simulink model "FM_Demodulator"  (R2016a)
settings: Solver=ode3  StartTime=0.0  StopTime=6  FixedStep=1/5000000  RelTol=1e-3
libraries: dsparch4 x4

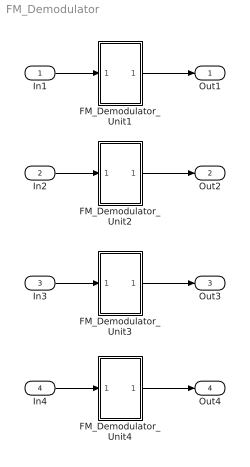
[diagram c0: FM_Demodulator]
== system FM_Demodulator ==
  In1 : Inport
  In2 : Inport  Port=2
  In3 : Inport  Port=3
  In4 : Inport  Port=4
  FM_Demodulator_Unit1 : Subsystem
  FM_Demodulator_Unit2 : Subsystem
  FM_Demodulator_Unit3 : Subsystem
  FM_Demodulator_Unit4 : Subsystem
  Out1 : Outport
  Out2 : Outport  Port=2
  Out3 : Outport  Port=3
  Out4 : Outport  Port=4
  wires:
  In1/1 -> FM_Demodulator_Unit1/1(In1)
  FM_Demodulator_Unit1/1(Out1) -> Out1/1
  In2/1 -> FM_Demodulator_Unit2/1(In1)
  FM_Demodulator_Unit2/1(Out1) -> Out2/1
  In3/1 -> FM_Demodulator_Unit3/1(In1)
  FM_Demodulator_Unit3/1(Out1) -> Out3/1
  In4/1 -> FM_Demodulator_Unit4/1(In1)
  FM_Demodulator_Unit4/1(Out1) -> Out4/1

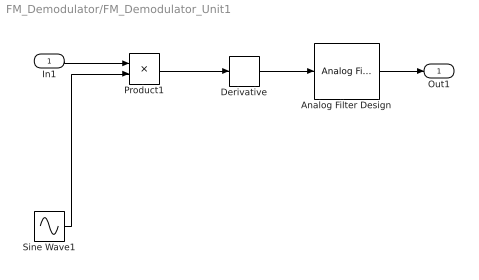
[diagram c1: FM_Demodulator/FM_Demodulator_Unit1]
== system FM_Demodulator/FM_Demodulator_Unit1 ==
  In1 : Inport
  Analog Filter Design : dsparch4/Analog Filter Design  method=Butterworth  filttype=Lowpass  N=10  Wlo=45000*2*pi  Whi=80  Rp=2  Rs=40
  Derivative : Derivative
  Product1 : Product
  Sine Wave1 : Sin  Frequency=500000*2*pi  Phase=-1.5*pi
  Out1 : Outport
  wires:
  Analog Filter Design/1 -> Out1/1
  Product1/1 -> Derivative/1
  Sine Wave1/1 -> Product1/2
  In1/1 -> Product1/1
  Derivative/1 -> Analog Filter Design/1

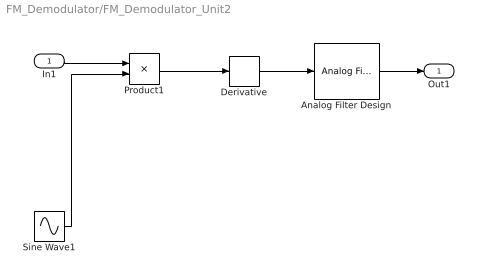
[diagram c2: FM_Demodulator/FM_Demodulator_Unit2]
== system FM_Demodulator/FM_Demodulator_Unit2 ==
  In1 : Inport
  Analog Filter Design : dsparch4/Analog Filter Design  method=Butterworth  filttype=Lowpass  N=10  Wlo=45000*2*pi  Whi=80  Rp=2  Rs=40
  Derivative : Derivative
  Product1 : Product
  Sine Wave1 : Sin  Frequency=500000*2*pi  Phase=-1.5*pi
  Out1 : Outport
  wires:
  Analog Filter Design/1 -> Out1/1
  Product1/1 -> Derivative/1
  Sine Wave1/1 -> Product1/2
  In1/1 -> Product1/1
  Derivative/1 -> Analog Filter Design/1

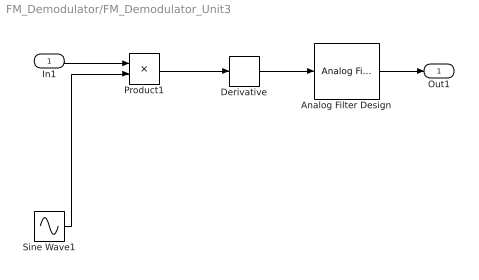
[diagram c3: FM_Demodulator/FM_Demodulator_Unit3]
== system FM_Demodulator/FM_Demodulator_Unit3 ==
  In1 : Inport
  Analog Filter Design : dsparch4/Analog Filter Design  method=Butterworth  filttype=Lowpass  N=10  Wlo=45000*2*pi  Whi=80  Rp=2  Rs=40
  Derivative : Derivative
  Product1 : Product
  Sine Wave1 : Sin  Frequency=500000*2*pi  Phase=-1.5*pi
  Out1 : Outport
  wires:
  Analog Filter Design/1 -> Out1/1
  Product1/1 -> Derivative/1
  Sine Wave1/1 -> Product1/2
  In1/1 -> Product1/1
  Derivative/1 -> Analog Filter Design/1

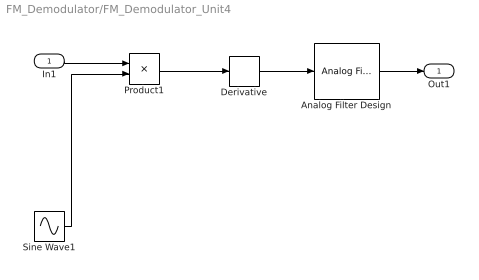
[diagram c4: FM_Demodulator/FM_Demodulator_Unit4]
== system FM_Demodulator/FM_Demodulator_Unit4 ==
  In1 : Inport
  Analog Filter Design : dsparch4/Analog Filter Design  method=Butterworth  filttype=Lowpass  N=10  Wlo=45000*2*pi  Whi=80  Rp=2  Rs=40
  Derivative : Derivative
  Product1 : Product
  Sine Wave1 : Sin  Frequency=500000*2*pi  Phase=-1.5*pi
  Out1 : Outport
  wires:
  Analog Filter Design/1 -> Out1/1
  Product1/1 -> Derivative/1
  Sine Wave1/1 -> Product1/2
  In1/1 -> Product1/1
  Derivative/1 -> Analog Filter Design/1
